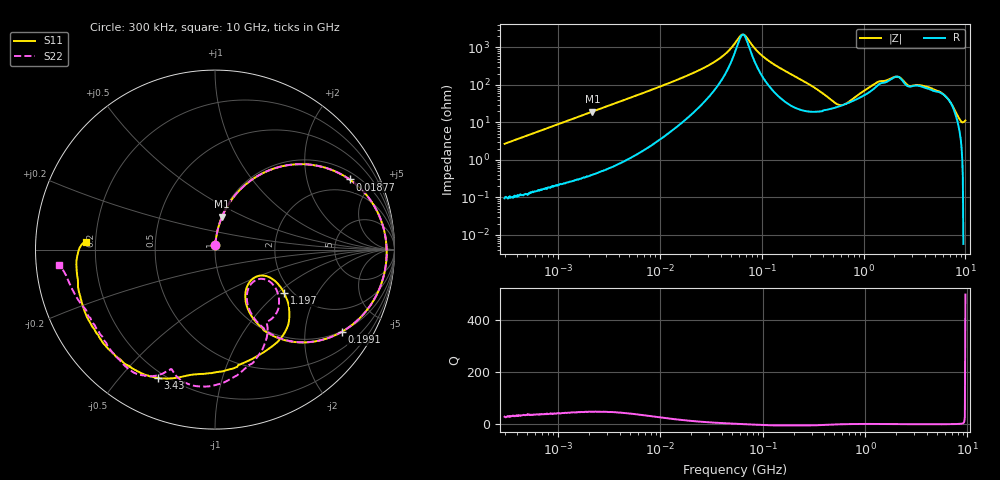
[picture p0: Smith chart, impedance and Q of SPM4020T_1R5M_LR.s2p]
! S-Parameter Data Generated by TDK Corporation
! Copyright(C) 2019 TDK Corporation.
! All Rights Reserved.
! TDK P/N: SPM4020T-1R5M-LR (Inductor)
! Property: L=1.5uH at 100kHz
! Size(LxWxT): 4.4x4.1x2mm
! Model Type: s2p (Touchstone File Format Version 1.0)
! Frequency: DC=Yes Start=0.3MHz Stop=10000MHz 802points Log-sweep
! Model Generated on Sep. 23, 2019
! Port Assignments:
!  1 ---@@@--- 2
! Applicable Conditions:
!  Temperature = 25 degC
!  DC Bias Current = 0 A
!  Small Signal Operation
! Terms and conditions regarding TDK Simulation Models
! (1)This simulation model is being provided solely for informational purposes. Please refer to the specifications of the products in terms of detailed characteristics of such products.
! (2)In no event shall TDK Corporation of any of its subsidiaries be liable for any loss or damage arising, directly or indirectly,
!  From any information contained in this simulation model, including, but not limited to loss or damages arising from any inaccuracies, omissions or errors in connection with such information.
! (3)Any and all copyrights on this simulation model are owned by TDK Corporation.
!  Duplication or redistribution of this simulation model without prior written permission from TDK Corporation is prohibited.
! (4)This simulation model is subject to any modification or change without any prior notice.
! (5)Neither TDK Corporation nor any of its subsidiaries shall make any warranty, express or implied,
!  Including but not limited to the correctness, implied warranties of merchantability and fitness for a particular purpose with respect to this simulation models.
! (6)The use of this simulation model shall be deemed to have consented to the terms and conditions hereof.
# Hz S MA R 50
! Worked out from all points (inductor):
!   801 points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, 300 kHz to 10 GHz, reference 50 ohm
!   read as one part in series: L = 1.42 uH near 318.3 kHz
!   highest Q = 48.1 at 2.179 MHz (marker M1), where L = 1.4 uH
!   self-resonance near 65.6 MHz
!   S11 on the Smith chart (normalised r, x): 300 kHz: 1.00, +0.05; 18.77 MHz: 1.32, +3.63; 199.1 MHz: 0.98, -3.09; 1.197 GHz: 1.82, -1.10; 3.43 GHz: 0.17, -0.64; 10 GHz: 0.16, +0.03
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300000  0.02658 86.6  0.9987 -1.5  0.9987 -1.6  0.02639 86.2
1713600  0.1487 80.2  0.9857 -8.6  0.9857 -8.6  0.1487 80.2
2178889  0.1874 77.9  0.9784 -10.9  0.9784 -10.9  0.1874 77.9
4796912  0.3851 65.8  0.9136 -22.8  0.9137 -22.8  0.3852 65.8
9671944  0.6412 47.6  0.7436 -40.2  0.7436 -40.2  0.6412 47.6
1.877128e7  0.8457 27.5  0.4747 -58.2  0.4747 -58.2  0.8457 27.5
3.642588e7  0.9383 10.4  0.2075 -68.3  0.2076 -68.3  0.9383 10.4
5.477226e7  0.9555 1.4  0.07401 -53.4  0.07403 -53.4  0.9555 1.4
6.736104e7  0.9567 -3.1  0.04418 8.6  0.0442 8.6  0.9567 -3.1
1.063884e8  0.9408 -13.7  0.1746 61.4  0.1746 61.4  0.9408 -13.7
1.990845e8  0.8416 -33.0  0.4351 49.0  0.4351 49.0  0.8416 -33.0
3.126428e8  0.6608 -50.7  0.6365 28.7  0.6365 28.7  0.6616 -50.5
5.911415e8  0.3011 -55.8  0.7568 -9.5  0.7568 -9.5  0.3096 -55.0
7.726947e8  0.2703 -34.9  0.7138 -26.8  0.7138 -26.8  0.2863 -36.1
1.196827e9  0.4536 -32.1  0.5236 -55.1  0.5237 -55.2  0.456 -38.5
1.767019e9  0.6381 -68.3  0.3375 -66.5  0.3375 -66.5  0.5803 -60.8
2.355454e9  0.6873 -90.9  0.2478 -54.6  0.2479 -54.6  0.7589 -91.1
2.720446e9  0.7074 -100.2  0.2858 -58.3  0.2858 -58.4  0.7388 -106.8
3.429941e9  0.7816 -113.9  0.2383 -71.0  0.2383 -71.0  0.746 -112.6
6.253087e9  0.8117 -138.2  0.1996 -93.1  0.1996 -93.2  0.7987 -140.2
8.211115e9  0.7851 -166.4  0.1619 -118.6  0.1622 -118.7  0.8283 -165.8
1e10  0.7184 176.7  0.123 -128.9  0.1229 -129.1  0.8736 -174.3
